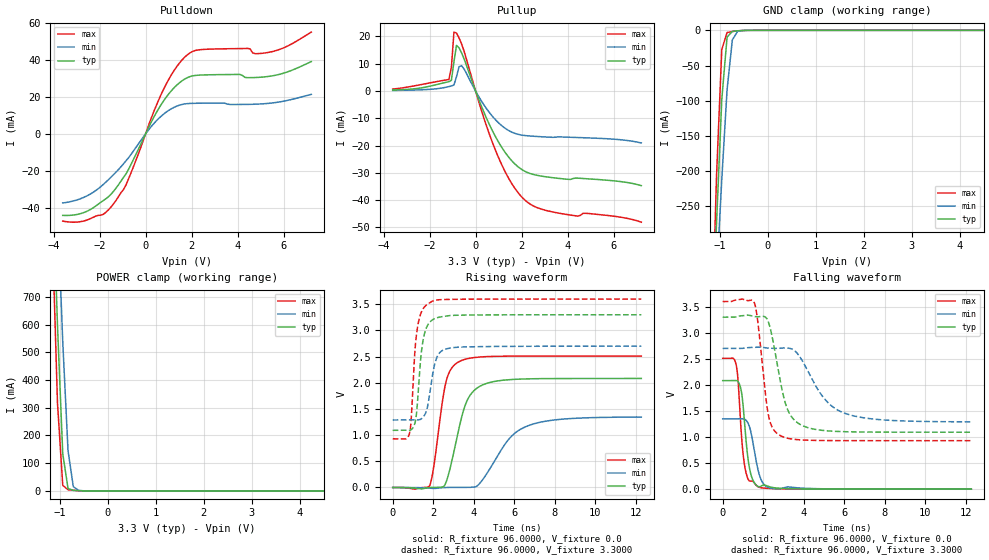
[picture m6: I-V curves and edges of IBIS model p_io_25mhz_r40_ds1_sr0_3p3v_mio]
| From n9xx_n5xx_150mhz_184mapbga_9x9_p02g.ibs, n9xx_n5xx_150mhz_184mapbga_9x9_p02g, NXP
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[Model] p_io_25mhz_r40_ds1_sr0_3p3v_mio
|   Model p_io_25mhz_r40_ds1_sr0_3p3v_mio
| This model was characterised for following simulation conditions:
| External (pad) voltage:
|   - Typ: 3.3V,   - Min: 2.7V,   - Max: 3.6V
| Library cells for typ/min/max conditions are connected as defined below:
|  pad - External Pad
|  ipp_do_lv - Core Input
|  ipp_obe_lv - Output Buffer Enable
|  IOGC - NC
|  REFH3V3 - REFH3V3
|  REFL3V3 - REFL3V3
|  ZI - NC
|  abut_ncal_vddio[1] - vddio
|  abut_ncal_vddio[2] - vddio
|  abut_ncal_vddio[3] - vssio
|  abut_ncal_vddio[4] - vddio
|  abut_ncal_vddio[5] - vddio
|  abut_ncal_vddio[6] - vssio
|  abut_pcal_vddio[1] - vssio
|  abut_pcal_vddio[2] - vssio
|  abut_pcal_vddio[3] - vddio
|  abut_pcal_vddio[4] - vssio
|  abut_pcal_vddio[5] - vssio
|  abut_pcal_vddio[6] - vddio
|  ipp_do_1p8v - ipp_do_1p8v
|  ipp_dse_lv - vdd_lv
|  ipp_eftd_lv - NC
|  ipp_ina_mux_vddio - NC
|  ipp_ina_mux_vddio[0] - NC
|  ipp_ina_mux_vddio[1] - NC
|  ipp_ina_r0_vddio - NC
|  ipp_ina_r0a_vddio - NC
|  ipp_ina_r0b_vddio - NC
|  ipp_ina_r0c_vddio - NC
|  ipp_ina_r0d_vddio - NC
|  ipp_ina_r0e_vddio - NC
|  ipp_ina_r0f_vddio - NC
|  ipp_ina_r300_vddio - NC
|  ipp_ina_r300a_vddio - NC
|  ipp_ina_r300b_vddio - NC
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Model_type I/O
Polarity   Non-Inverting
Enable   Active-High
Vinl =   0.9900V
Vinh =   2.3100V
Vmeas =  1.6500V
Cref =   30.0000pF
Rref =   1.0000M
Vref =   3.3000V
C_comp   1.6860pF   1.6265pF   1.7672pF
|C_comp_pullup   0.5953pF   0.6263pF   0.5740pF
|C_comp_pulldown   0.8303pF   0.8787pF   0.7927pF
[Model Spec]
| variable   typ   min   max
Vinh   2.3100V   1.8900V   2.5200V
Vinl   0.9900V   0.8100V   1.0800V
[Temperature Range]   25.0000   0.1250k   -40.0000
[Voltage Range]   3.3000V   2.7000V   3.6000V
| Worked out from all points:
|   slope of the pulldown table from 0 to 0.495 V, typ, clamps not added: 40.9 ohm
|   slope of the pullup table from 0 to 0.495 V, typ, clamps not added: 47.8 ohm
|   GND clamp passes 1 mA (typ) near -0.67 V on its own axis
|   POWER clamp passes 1 mA (typ) near -0.62 V on its own axis
|   rising waveform, R_fixture 96.0000, V_fixture 0.0: 20-80 % time 814ps typ, 1.51ns min, 558ps max; typ from 0 V to 2.08 V
|   rising waveform, R_fixture 96.0000, V_fixture 3.3000: 20-80 % time 317ps typ, 384ps min, 288ps max; typ from 1.09 V to 3.3 V
|   falling waveform, R_fixture 96.0000, V_fixture 0.0: 20-80 % time 324ps typ, 412ps min, 289ps max; typ from 2.08 V to 0 V
|   falling waveform, R_fixture 96.0000, V_fixture 3.3000: 20-80 % time 720ps typ, 1.46ns min, 458ps max; typ from 3.3 V to 1.09 V
[Pulldown]
|Voltage   I(typ)   I(min)   I(max)
-3.6V     -44.24mA   -37.49mA   -47.33mA
-2.5V     -41.72mA   -33.35mA   -46.54mA
-1.84V    -36.2mA    -27.49mA   -43.67mA
-1.4V     -31.29mA   -22.21mA   -38.12mA
-850mV    -21.76mA   -14.6mA    -27.7mA
800mV     18.19mA    10.89mA    24.63mA
1.35V     26.39mA    15.02mA    36.42mA
1.9V      30.94mA    16.48mA    43.69mA
4.43V     30.49mA    15.99mA    46.36mA
4.76V     30.57mA    16.1mA     43.49mA
5.31V     31.12mA    16.52mA    44.14mA
7.2V      39.23mA    21.44mA    55.22mA
[Pullup]
|Voltage   I(typ)   I(min)   I(max)
-3.6V     375.6uA    207.3uA    723.2uA
-1.16V    3.421mA    1.609mA    4.222mA
-1.05V    3.932mA    1.826mA    8.69mA
-940mV    10.66mA    2.21mA     21.59mA
-830mV    16.71mA    5.23mA     21.25mA
-720mV    15.83mA    8.864mA    19.49mA
-610mV    14.01mA    9.303mA    17.31mA
820mV     -16.02mA   -10.13mA   -20.77mA
1.48V     -24.67mA   -14.68mA   -32.64mA
2.03V     -28.89mA   -16.19mA   -39.05mA
3.35V     -31.77mA   -16.98mA   -44.33mA
7.2V      -34.69mA   -19.04mA   -48.08mA
[GND_clamp]
|Voltage   I(typ)   I(min)   I(max)
-3.6V     -5.343A    -4.159A    -6.913A
-1.18V    -470.5mA   -501mA     -462.9mA
-1.07V    -274.4mA   -353mA     -207.6mA
-960mV    -98.09mA   -211.4mA   -27.2mA
-850mV    -9.59mA    -84.32mA   -3.159mA
-740mV    -1.542mA   -13.52mA   -1.688mA
-630mV    -656uA     -1.44mA    -722.1uA
-300mV    -859.4nA   -5.611uA   -163.9nA
7.2V      0A         0A         0A
[POWER_clamp]
|Voltage   I(typ)   I(min)   I(max)
-3.6V     14.48A     12.95A     16.35A
-1.16V    1.177A     1.535A     951.2mA
-1.05V    598.4mA    1.032A     318mA
-940mV    134.2mA    537.3mA    20.05mA
-830mV    8.719mA    145.4mA    4.267mA
-720mV    2.135mA    15.38mA    2.236mA
-610mV    852.8uA    1.854mA    844.7uA
7.2V      0A         0A         0A
[Ramp]
| variable   typ   min   max
dV/dt_r  1.2496/0.8139n   0.8078/1.5136n   1.5064/0.5575n
dV/dt_f  1.3245/0.7197n   0.8451/1.4616n   1.6019/0.4585n
R_load = 96.0000
[Rising Waveform]
R_fixture= 96.0000
V_fixture= 0.0
V_fixture_min= 0.0
V_fixture_max= 0.0
|time   V(typ)   V(min)   V(max)
0s        3.106nV    104.7nV    10.55nV
1.819ns   -1.009mV   -14.1mV    31.42mV
2.018ns   1.375mV    -17.5mV    376.2mV
2.636ns   104.4mV    -182.2uV   2.027V
3.288ns   1.16V      1.223mV    2.407V
3.819ns   1.762V     2.672mV    2.471V
4.739ns   2.001V     322.3mV    2.502V
5.778ns   2.061V     944.9mV    2.509V
6.814ns   2.077V     1.198V     2.51V
12.27ns   2.083V     1.346V     2.511V
[Rising Waveform]
R_fixture= 96.0000
V_fixture= 3.3000
V_fixture_min= 2.7000
V_fixture_max= 3.6000
|time   V(typ)   V(min)   V(max)
0s        1.093V     1.289V     930.2mV
830.6ps   1.092V     1.289V     1.035V
914.2ps   1.105V     1.289V     1.312V
1.072ns   1.199V     1.289V     2.468V
1.234ns   1.678V     1.29V      3.083V
1.486ns   2.785V     1.337V     3.404V
1.942ns   3.198V     2.099V     3.557V
2.254ns   3.25V      2.542V     3.586V
2.875ns   3.287V     2.666V     3.594V
12.27ns   3.3V       2.7V       3.6V
[Falling Waveform]
R_fixture= 96.0000
V_fixture= 0.0
V_fixture_min= 0.0
V_fixture_max= 0.0
|time   V(typ)   V(min)   V(max)
0s        2.083V     1.349V     2.511V
630.9ps   2.085V     1.349V     2.434V
739.9ps   2.071V     1.349V     2.171V
852.1ps   1.987V     1.349V     1.475V
987.4ps   1.68V      1.351V     742.2mV
1.153ns   928.9mV    1.322V     312.1mV
1.384ns   294.2mV    1.109V     155.1mV
1.754ns   49.32mV    353.9mV    44.66mV
2.577ns   24.88mV    9.146mV    8.565mV
12.27ns   246.7nV    17.14uV    31.95nV
[Falling Waveform]
R_fixture= 96.0000
V_fixture= 3.3000
V_fixture_min= 2.7000
V_fixture_max= 3.6000
|time   V(typ)   V(min)   V(max)
0s        3.3V       2.7V       3.6V
1.558ns   3.314V     2.722V     3.581V
1.733ns   3.306V     2.726V     3.214V
2.249ns   3.214V     2.707V     1.437V
2.845ns   2.068V     2.705V     1.026V
3.186ns   1.542V     2.709V     978.1mV
3.616ns   1.297V     2.634V     952.4mV
4.992ns   1.125V     1.748V     933.2mV
5.93ns    1.104V     1.471V     931.1mV
12.27ns   1.093V     1.291V     930.2mV
